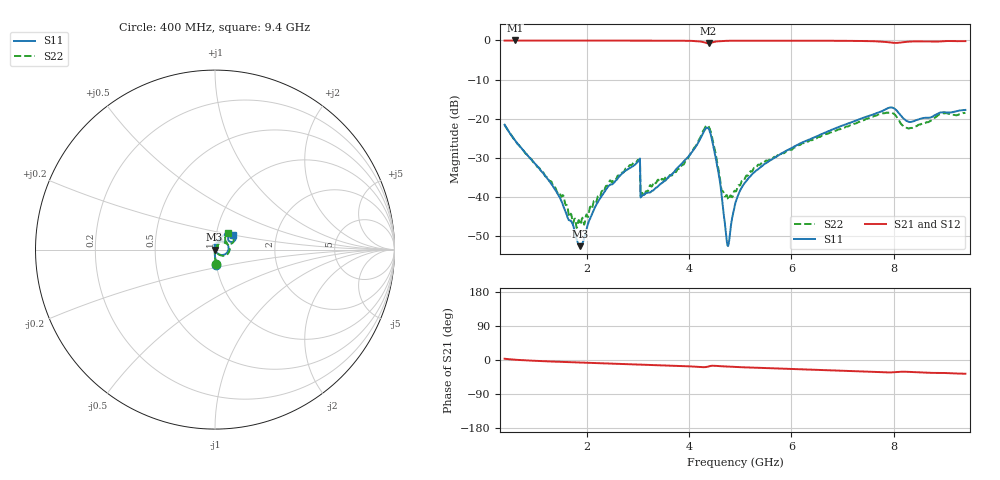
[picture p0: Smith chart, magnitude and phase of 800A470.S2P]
!  American Technical Ceramics  Date:  9/12/2007
!  One Norden Lane
!  Huntington Station,  NY.  11746-2102
!  Tel:  (631) 622-4700  Fax:  (631) 622-4748
!  Part Number  800A470  Mounting Orientation: Vertical
!  Description: Ultra Low ESR Microwave capacitors
!  Application: Coupling, Bypass, Tuning, DC Block
!  Filters, Matching
# GHZ S DB R 50
! Freq  |S11|  S11 Ph  |S21|  S21 Ph  |S12|  S12 Ph  |S22|  S22 Ph
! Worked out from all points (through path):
!   801 points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, 400 MHz to 9.4 GHz, reference 50 ohm
!   highest |S21| = -0.02 dB at 603 MHz (marker M1); lowest = -0.8 dB at 4.383 GHz (marker M2)
!   group delay of S21, straight-line fit = 11.4 ps
!   lowest |S11| = -52.6 dB at 1.874 GHz (marker M3), VSWR 1.00, Z = 49.8 + j0.0481 ohm
!   |S11| at or under -10 dB: start of sweep to end of sweep
!   |S22| runs from -47.9 to -18.4 dB; largest |S21 - S12| = 0.003
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0.4  -21.55 -86.3  -0.04 3.3  -0.05 3.3  -21.60 -86.2
0.603  -25.53 -88.8  -0.02 0.8  -0.03 0.8  -25.48 -87.8
1.368  -37.77 -99.0  -0.02 -4.2  -0.03 -4.2  -37.52 -80.7
1.874  -52.58 168.1  -0.04 -6.7  -0.04 -6.6  -46.97 -13.9
1.908  -52.30 148.7  -0.04 -6.9  -0.04 -6.8  -45.64 1.1
2.211  -41.55 102.2  -0.04 -8.3  -0.04 -8.2  -40.16 45.4
2.751  -33.39 90.7  -0.06 -10.8  -0.06 -10.7  -33.00 59.2
2.999  -31.09 93.2  -0.06 -11.8  -0.07 -11.8  -30.59 58.2
3.1  -39.55 89.8  -0.06 -12.2  -0.06 -12.1  -39.27 38.4
3.404  -37.16 90.0  -0.07 -13.6  -0.07 -13.5  -35.62 47.2
3.854  -31.57 83.2  -0.09 -15.8  -0.09 -15.8  -32.05 59.9
4.383  -22.54 -2.3  -0.76 -17.0  -0.76 -16.9  -22.00 -8.5
4.563  -32.75 -58.8  -0.24 -15.9  -0.24 -15.8  -32.05 -53.4
4.664  -42.74 -61.7  -0.16 -16.7  -0.16 -16.6  -38.51 -28.1
4.743  -51.63 -15.2  -0.11 -17.3  -0.11 -17.2  -39.57 -4.4
4.788  -50.98 46.3  -0.10 -17.6  -0.10 -17.6  -40.43 13.2
4.9  -41.99 79.2  -0.09 -18.3  -0.09 -18.3  -38.45 34.5
5.271  -33.77 78.5  -0.08 -20.3  -0.08 -20.2  -32.57 58.2
6.408  -25.01 68.6  -0.09 -25.5  -0.08 -25.4  -25.49 59.0
7.904  -17.23 40.8  -0.49 -32.8  -0.48 -32.8  -18.47 34.1
8.309  -20.85 32.9  -0.31 -31.5  -0.30 -31.4  -22.47 37.0
9.4  -17.77 40.4  -0.19 -36.2  -0.18 -36.1  -18.47 52.3
